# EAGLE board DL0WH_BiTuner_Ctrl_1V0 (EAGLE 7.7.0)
DL0WH Antenna BiTuner
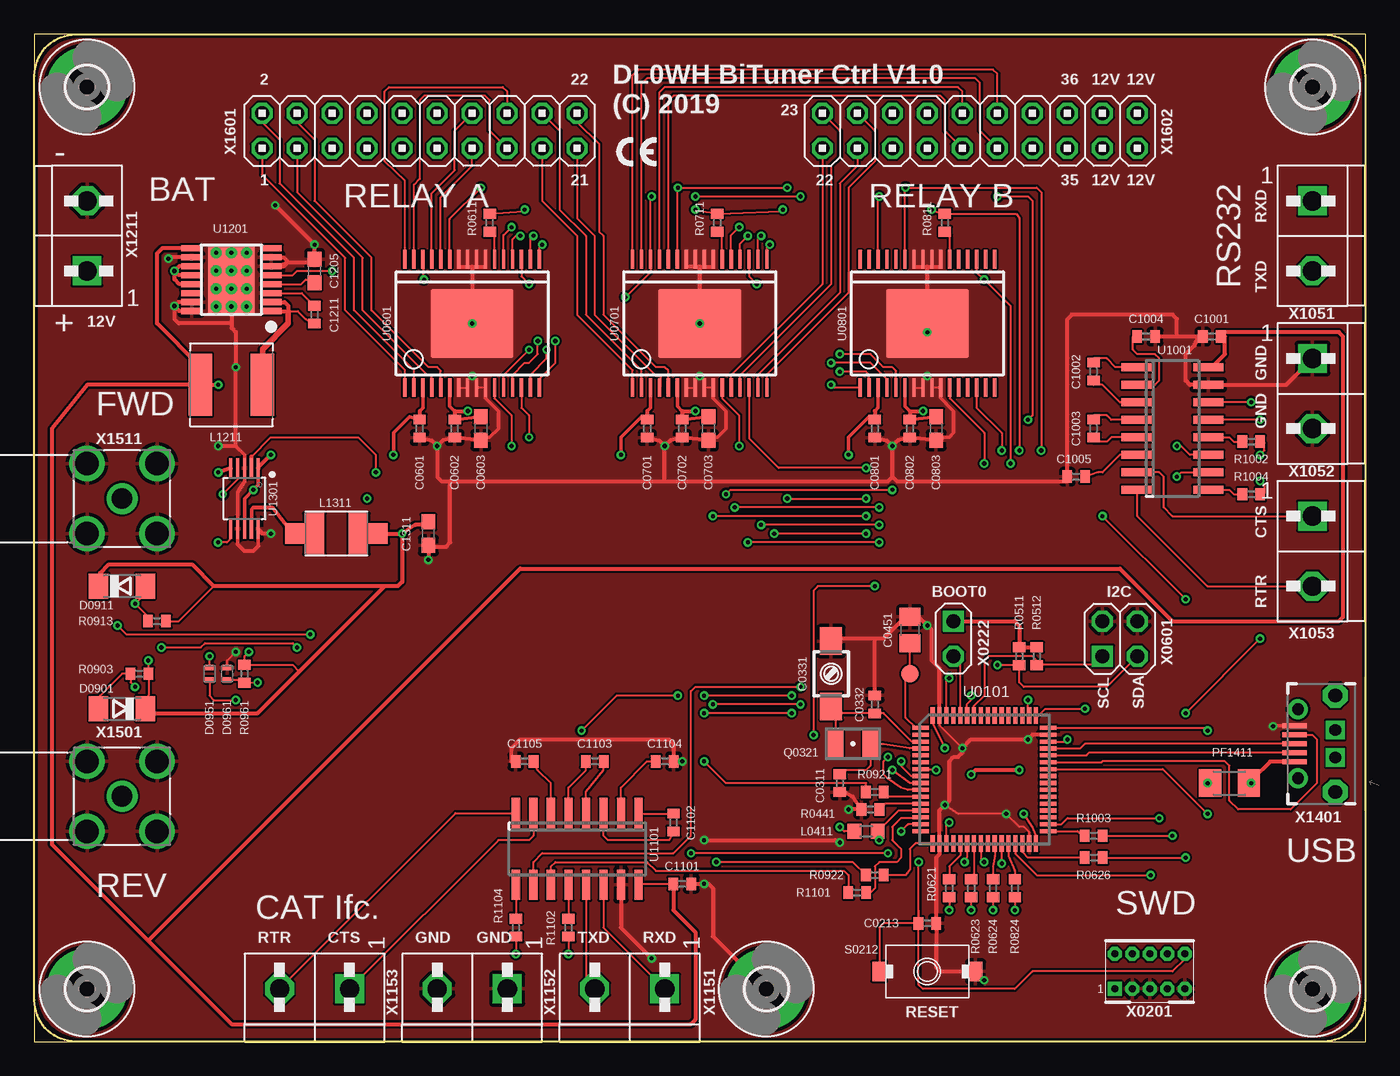
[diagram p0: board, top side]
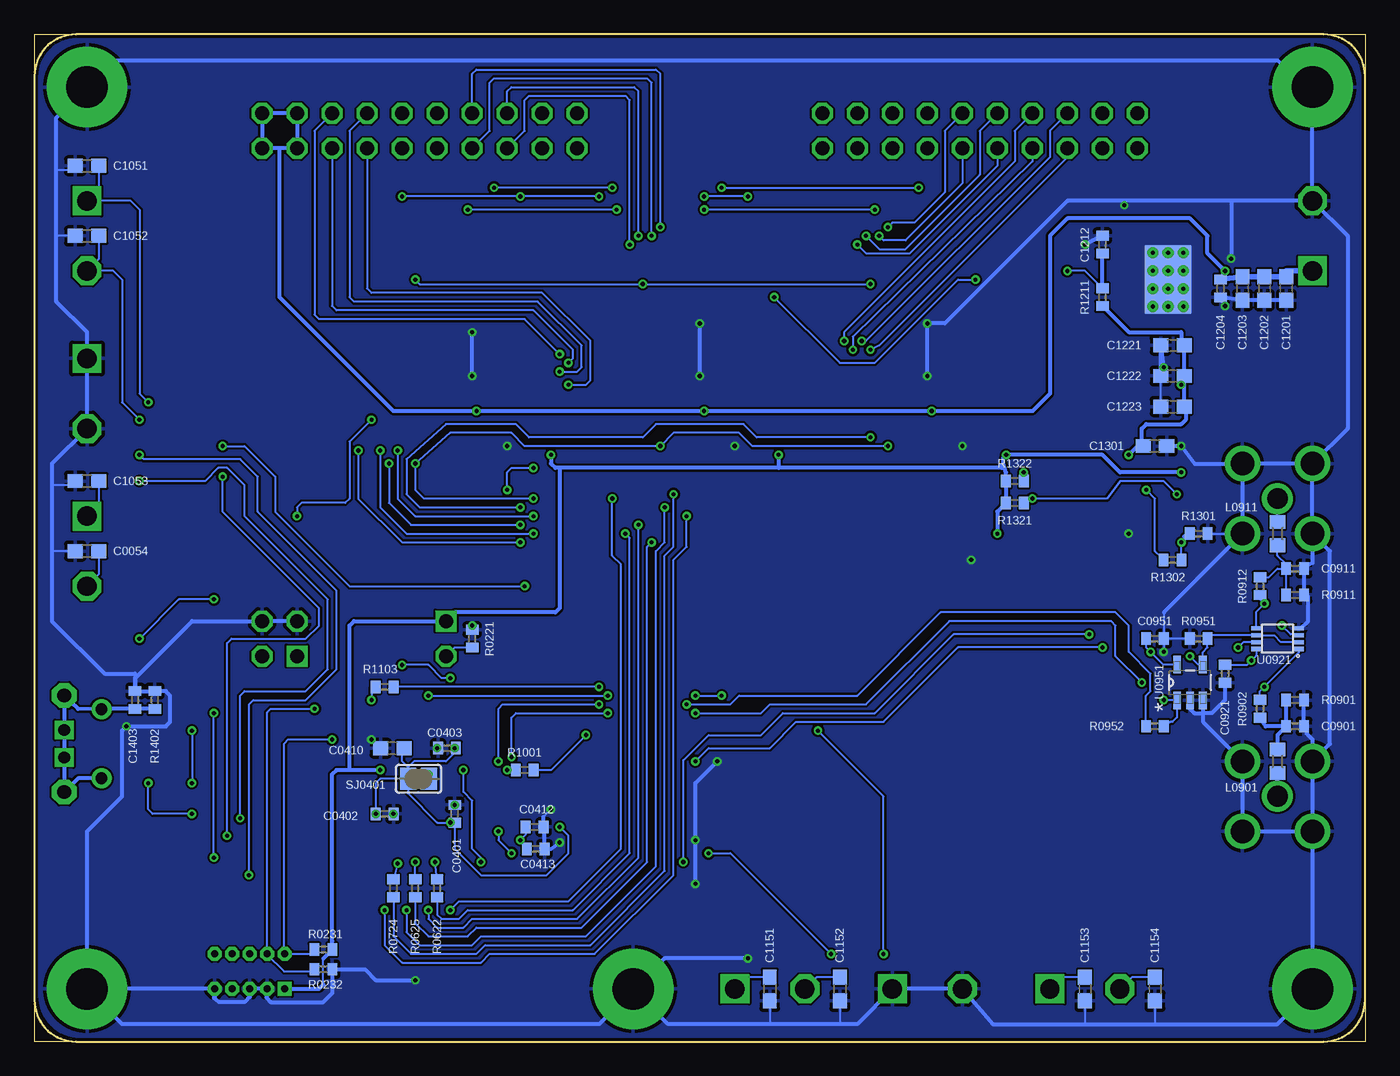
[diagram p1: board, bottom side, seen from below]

Size 96.52 x 73.03 mm. Coordinates in mm from the lower left corner, seen from the top.
Outline: 0,0 96.52,0 96.52,73.03 0,73.03 0,0
Copper layers (1*16): Top 0.035mm / dielectric 1.5mm / Bottom 0.035mm
Design rules "DL0WH_BiTuner_MCU_1V0": minimum track width 6mil, minimum drill 0.3mm, track to track 6mil, track to pad 6mil, pad to pad 6mil, via to via 6mil, smd to smd 0mil, copper to edge 10mil, drill to drill 10mil, minimum pad ring 10mil, minimum via ring 6mil, stop-mask expansion 2mil, vias tented up to drill 25mil, thermal gap 10mil
Net classes: 1 pwr_relay: width 1.5 mm, clearance 0.5 mm; 2 pwr_ttl: width 0.75 mm, clearance 0.5 mm; 3 usb_pair: width 0.254 mm, clearance 0.152 mm; 4 pwrA5: width 0.4 mm; 5 single50R: width 0.838 mm, clearance 0.152 mm
Milling: 8 lines

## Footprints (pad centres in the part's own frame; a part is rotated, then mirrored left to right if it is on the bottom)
C0603 = smd 1.1 x 1: 1 -0.85,0; 2 0.85,0
C0402 = smd 0.7 x 0.9: 1 -0.65,0; 2 0.65,0
3MM2_X_2MM5 = smd 2 x 1.6: + -2.365,0; - 2.365,0
C0805 = smd 1.3 x 1.5: 1 -0.95,0; 2 0.95,0
SOD80C = smd 1.4 x 1.8: A 1.7,0; C -1.7,0
SOD923 = smd 0.4 x 0.6: A 0.45,0; C -0.45,0
3,0-PAD = drill 3 pad 5.842: B3,0 0,0
L0603 = smd 1 x 1.1: 1 -0.85,0; 2 0.85,0
L_6.00MM_X_6.00MM = smd 1.7 x 4.5: 1 -2.25,0; 2 2.25,0
L_4.50MM_X_3.20MM = smd 1.5 x 3: 1 -1.6,0; 2 1.6,0 | smd 2 x 1.5: 3 -2.75,0; 4 2.75,0
M1206 = smd 1.6 x 2: 1 -1.4,0; 2 1.4,0
ABS07 = smd 1.1 x 1.9: 1 -1.25,0; 2 1.25,0
R0402 = smd 0.7 x 0.9: 1 -0.65,0; 2 0.65,0
KSR223G_SMD_1POL = smd 1 x 1.4: 1 -3.5,0; 2 3.5,0
SJ = smd 1.168 x 1.6: 1 -0.762,0; 2 0.762,0
B1,27 = smd 1.27 x 1.27: TP 0,0
LQFP64 = smd 0.3 x 1.2: 1 -3.7,-4.3; 2 -3.2,-4.3; 3 -2.7,-4.3; 4 -2.2,-4.3; 5 -1.7,-4.3; 6 -1.2,-4.3; 7 -0.7,-4.3; 8 -0.2,-4.3; 9 0.3,-4.3; 10 0.8,-4.3; 11 1.3,-4.3; 12 1.8,-4.3; 13 2.3,-4.3; 14 2.8,-4.3; 15 3.3,-4.3; 16 3.8,-4.3; 33 3.8,4.95; 34 3.3,4.95; 35 2.8,4.95; 36 2.3,4.95; 37 1.8,4.95; 38 1.3,4.95; 39 0.8,4.95; 40 0.3,4.95; 41 -0.2,4.95; 42 -0.7,4.95; 43 -1.2,4.95; 44 -1.7,4.95; 45 -2.2,4.95; 46 -2.7,4.95; 47 -3.2,4.95; 48 -3.7,4.95 | smd 1.2 x 0.3: 17 4.675,-3.425; 18 4.675,-2.925; 19 4.675,-2.425; 20 4.675,-1.925; 21 4.675,-1.425; 22 4.675,-0.925; 23 4.675,-0.425; 24 4.675,0.075; 25 4.675,0.575; 26 4.675,1.075; 27 4.675,1.575; 28 4.675,2.075; 29 4.675,2.575; 30 4.675,3.075; 31 4.675,3.575; 32 4.675,4.075; 49 -4.575,4.075; 50 -4.575,3.575; 51 -4.575,3.075; 52 -4.575,2.575; 53 -4.575,2.075; 54 -4.575,1.575; 55 -4.575,1.075; 56 -4.575,0.575; 57 -4.575,0.075; 58 -4.575,-0.425; 59 -4.575,-0.925; 60 -4.575,-1.425; 61 -4.575,-1.925; 62 -4.575,-2.425; 63 -4.575,-2.925; 64 -4.575,-3.425
SOICW32 = smd 0.25 x 1.3: 1 -4.875,-4.65; 2 -4.225,-4.65; 3 -3.575,-4.65; 4 -2.925,-4.65; 5 -2.275,-4.65; 6 -1.625,-4.65; 7 -0.975,-4.65; 8 -0.325,-4.65; 9 0.325,-4.65; 10 0.975,-4.65; 11 1.625,-4.65; 12 2.275,-4.65; 13 2.925,-4.65; 14 3.575,-4.65; 15 4.225,-4.65; 16 4.875,-4.65; 17 4.875,4.65; 18 4.225,4.65; 19 3.575,4.65; 20 2.925,4.65; 21 2.275,4.65; 22 1.625,4.65; 23 0.975,4.65; 24 0.325,4.65; 25 -0.325,4.65; 26 -0.975,4.65; 27 -1.625,4.65; 28 -2.275,4.65; 29 -2.925,4.65; 30 -3.575,4.65; 31 -4.225,4.65; 32 -4.875,4.65 | smd 6 x 5: 33 0,0
R-PDSO-G8 = smd 0.25 x 0.75: 1 -0.75,-1.55; 2 -0.25,-1.55; 3 0.25,-1.55; 4 0.75,-1.55; 5 0.75,1.55; 6 0.25,1.55; 7 -0.25,1.55; 8 -0.75,1.55
SOT-23-5 = smd 1.27 x 0.559: 1 -1.295,0.94; 2 -1.295,0; 3 -1.295,-0.94; 4 1.295,-0.94; 5 1.295,0.94
SOIC16N = smd 0.6 x 2.2: 1 -4.445,-2.6; 2 -3.175,-2.6; 3 -1.905,-2.6; 4 -0.635,-2.6; 5 0.635,-2.6; 6 1.905,-2.6; 7 3.175,-2.6; 8 4.445,-2.6; 9 4.445,2.6; 10 3.175,2.6; 11 1.905,2.6; 12 0.635,2.6; 13 -0.635,2.6; 14 -1.905,2.6; 15 -3.175,2.6; 16 -4.445,2.6
HTSSOP16 = smd 0.45 x 1.5: 1 -2.275,-2.9; 2 -1.625,-2.9; 3 -0.975,-2.9; 4 -0.325,-2.9; 5 0.325,-2.9; 6 0.975,-2.9; 7 1.625,-2.9; 8 2.275,-2.9; 9 2.275,2.9; 10 1.625,2.9; 11 0.975,2.9; 12 0.325,2.9; 13 -0.325,2.9; 14 -0.975,2.9; 15 -1.625,2.9; 16 -2.275,2.9 | drill 0.305 pad 0.61: PAD 0.65,0; PAD3 -0.65,0; PAD4 -1.95,0; PAD5 1.95,0; PAD6 1.95,1.1; PAD7 1.95,-1.1; PAD8 0.65,1.1; PAD9 0.65,-1.1; PAD10 -0.65,1.1; PAD11 -0.65,-1.1; PAD12 -1.95,1.1; PAD13 -1.95,-1.1 | smd 5 x 3.4: PAD1 0,0 | smd 5 x 3.4 bottom: PAD2 0,0
S-PDSO-G10 = smd 0.3 x 1.45: 1 -1,-2.2; 2 -0.5,-2.2; 3 0,-2.2; 4 0.5,-2.2; 5 1,-2.2; 6 1,2.2; 7 0.5,2.2; 8 0,2.2; 9 -0.5,2.2; 10 -1,2.2
2X05_SHROUDED_1MM27 = drill 0.508 pad 0.813 square: 1 -2.54,-1.27 | drill 0.508 pad 0.813 octagon: 2 -2.54,1.27; 3 -1.27,-1.27; 4 -1.27,1.27; 5 0,-1.27; 6 0,1.27; 7 1.27,-1.27; 8 1.27,1.27; 9 2.54,-1.27; 10 2.54,1.27
1X02 = drill 1.016 square: 1 0,0 | drill 1.016 octagon: 2 0,2.54
2X02 = drill 1.016 square: 1 -1.27,-1.27 | drill 1.016 octagon: 2 -1.27,1.27; 3 1.27,-1.27; 4 1.27,1.27
WIRE-TO-BOARD_5MM08_1X02 = drill 1.4 square: 1 0,2.54 | drill 1.4 octagon: 2 0,-2.54
USB-B-MICRO-SMD_MOLEX-105017-0001 = smd 0.35 x 1.8: D+ 0,4.4; D- -0.65,4.4; GND 1.3,4.4; ID 0.65,4.4; VBUS -1.3,4.4 | drill 0.85 pad 1.45: JSHIELD -2.5,4.15; JSHIELD@2 2.5,4.15 | drill 1 pad 1.8 octagon: JSHIELD@3 -3.5,1.45; JSHIELD@6 3.5,1.45 | drill 0.85 square: JSHIELD@4 -1,1.45; JSHIELD@5 1,1.45
SMA_SMT_AMPHENOL_901-143 = drill 1.499: 1 0,0 | drill 1.702: 2 -2.54,2.54; 3 -2.54,-2.54; 4 2.54,-2.54; 5 2.54,2.54
2X10 = drill 1.016 octagon: 1 -11.43,-1.27; 2 -11.43,1.27; 3 -8.89,-1.27; 4 -8.89,1.27; 5 -6.35,-1.27; 6 -6.35,1.27; 7 -3.81,-1.27; 8 -3.81,1.27; 9 -1.27,-1.27; 10 -1.27,1.27; 11 1.27,-1.27; 12 1.27,1.27; 13 3.81,-1.27; 14 3.81,1.27; 15 6.35,-1.27; 16 6.35,1.27; 17 8.89,-1.27; 18 8.89,1.27; 19 11.43,-1.27; 20 11.43,1.27

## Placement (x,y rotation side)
C0054  10nF  [C0603]  92.71,35.56 180 bottom
C0213  100nF  [C0402]  64.77,8.57 0 top
C0311  18pF  [C0402]  58.42,18.73 270 top
C0331  JR200  [3MM2_X_2MM5]  57.78,26.67 270 top
C0332  8.2pF  [C0402]  60.96,24.45 90 top
C0401  100nF  [C0402]  66.04,16.51 90 bottom
C0402  100nF  [C0402]  71.12,16.51 0 bottom
C0403  100nF  [C0402]  66.6,21.27 180 bottom
C0410  4.7uF  [C0603]  70.56,21.27 180 bottom
C0412  10nF  [C0402]  60.25,15.56 0 bottom
C0413  1uF  [C0402]  60.17,13.97 0 bottom
C0451  47uF  [C0805]  63.5,29.84 90 top
C0601  100nF  [C0402]  27.94,44.45 90 top
C0602  100nF  [C0402]  30.48,44.45 270 top
C0603  22uF  [C0603]  32.38,44.45 270 top
C0701  100nF  [C0402]  44.45,44.45 90 top
C0702  100nF  [C0402]  46.99,44.45 270 top
C0703  22uF  [C0603]  48.9,44.45 270 top
C0801  100nF  [C0402]  60.96,44.45 90 top
C0802  100nF  [C0402]  63.5,44.45 270 top
C0803  22uF  [C0603]  65.41,44.45 270 top
C0901  10nF  [C0402]  5.08,22.86 0 bottom
C0911  10nF  [C0402]  5.08,34.29 0 bottom
C0921  100nF  [C0402]  10.16,26.67 270 bottom
C0951  100nF  [C0402]  15.24,29.21 0 bottom
C1001  1uF  [C0402]  85.41,51.12 180 top
C1002  1uF  [C0402]  76.83,48.58 270 top
C1003  1uF  [C0402]  76.83,44.45 270 top
C1004  1uF  [C0402]  80.64,51.12 0 top
C1005  1uF  [C0402]  75.56,40.96 180 top
C1051  10nF  [C0603]  92.71,63.5 180 bottom
C1052  10nF  [C0603]  92.71,58.42 180 bottom
C1053  10nF  [C0603]  92.71,40.64 180 bottom
C1101  1uF  [C0402]  46.99,11.43 0 top
C1102  1uF  [C0402]  46.35,15.88 270 top
C1103  1uF  [C0402]  40.64,20.32 180 top
C1104  1uF  [C0402]  45.72,20.32 0 top
C1105  1uF  [C0402]  35.56,20.32 180 top
C1151  10nF  [C0603]  43.18,3.81 270 bottom
C1152  10nF  [C0603]  38.1,3.81 270 bottom
C1153  10nF  [C0603]  20.32,3.81 270 bottom
C1154  10nF  [C0603]  15.24,3.81 270 bottom
C1201  10uF  [C0603]  5.71,54.61 270 bottom
C1202  10uF  [C0603]  7.3,54.61 270 bottom
C1203  10uF  [C0603]  8.89,54.61 270 bottom
C1204  10nF  [C0402]  10.48,54.61 270 bottom
C1205  3.3uF  [C0603]  20.32,55.88 270 top
C1211  0.47uF  [C0402]  20.32,52.7 90 top
C1212  100nF  [C0402]  19.05,57.78 90 bottom
C1221  22uF  [C0603]  13.97,50.48 180 bottom
C1222  22uF  [C0603]  13.97,48.26 180 bottom
C1223  22uF  [C0603]  13.97,46.04 180 bottom
C1301  22uF  [C0603]  15.24,43.18 0 bottom
C1311  22uF  [C0603]  28.57,36.83 270 top
C1403  1nF  [C0402]  89.22,24.77 270 bottom
D0901  CRS08  [SOD80C]  6.35,24.13 180 top
D0911  CRS08  [SOD80C]  6.35,33.02 0 top
D0951  CMAD6001  [SOD923]  12.7,26.67 90 top
D0961  CMAD6001  [SOD923]  13.97,26.67 270 top
H1711  MOUNT-PAD-ROUND3.0  [3,0-PAD]  3.81,3.81 0 top
H1721  MOUNT-PAD-ROUND3.0  [3,0-PAD]  53.09,3.81 0 top
H1731  MOUNT-PAD-ROUND3.0  [3,0-PAD]  92.71,3.81 0 top
H1751  MOUNT-PAD-ROUND3.0  [3,0-PAD]  3.81,69.22 0 top
H1761  MOUNT-PAD-ROUND3.0  [3,0-PAD]  92.71,69.22 0 top
L0411  10uH  [L0603]  60.33,15.24 0 top
L0901  10uH  [L0603]  6.35,20.32 270 bottom
L0911  10uH  [L0603]  6.35,36.83 90 bottom
L1211  2.2uH  [L_6.00MM_X_6.00MM]  14.29,47.62 0 top
L1311  10uH  [L_4.50MM_X_3.20MM]  21.91,36.83 180 top
PF1411  1.1A/2.2A  [M1206]  86.68,18.73 180 top
Q0321  ABS07-32.768KHZ  [ABS07]  59.37,21.59 180 top
R0221  33kR  [R0402]  64.77,29.21 270 bottom
R0231  220kR  [R0402]  75.56,6.67 0 bottom
R0232  220kR  [R0402]  75.56,5.24 180 bottom
R0441  0R  [R0402]  60.64,16.83 0 top
R0511  1kR  [R0402]  71.44,27.94 90 top
R0512  1kR  [R0402]  72.71,27.94 90 top
R0611  47R  [R0402]  33.02,59.37 270 top
R0621  47R  [R0402]  66.36,11.11 270 top
R0622  0R  [R0402]  67.31,11.11 270 bottom
R0623  47R  [R0402]  67.94,11.11 270 top
R0624  47R  [R0402]  69.53,11.11 270 top
R0625  47R  [R0402]  68.9,11.11 270 bottom
R0626  47R  [R0402]  76.83,13.34 0 top
R0711  47R  [R0402]  49.53,59.37 270 top
R0724  47R  [R0402]  70.48,11.11 270 bottom
R0811  47R  [R0402]  66.04,59.37 270 top
R0824  47R  [R0402]  71.12,11.11 270 top
R0901  1kR  [R0402]  5.08,24.77 180 bottom
R0902  15kR  [R0402]  7.62,24.13 90 bottom
R0903  100kR  [R0402]  7.62,26.67 0 top
R0911  1kR  [R0402]  5.08,32.38 180 bottom
R0912  15kR  [R0402]  7.62,33.02 270 bottom
R0913  100kR  [R0402]  8.89,30.48 0 top
R0921  47R  [R0402]  60.96,18.1 180 top
R0922  47R  [R0402]  60.96,12.06 180 top
R0951  1MR  [R0402]  12.06,29.21 0 bottom
R0952  47R  [R0402]  15.24,22.86 180 bottom
R0961  10kR  [R0402]  15.24,26.67 270 top
R1001  47R  [R0402]  60.96,19.68 0 bottom
R1002  47R  [R0402]  88.27,43.5 180 top
R1003  47R  [R0402]  76.83,14.92 0 top
R1004  47R  [R0402]  88.27,39.69 180 top
R1101  47R  [R0402]  59.69,10.79 180 top
R1102  47R  [R0402]  38.73,8.26 90 top
R1103  47R  [R0402]  71.12,25.72 0 bottom
R1104  47R  [R0402]  34.92,8.26 90 top
R1211  3R  [R0402]  19.05,53.98 270 bottom
R1301  100kR  [R0402]  12.06,36.83 180 bottom
R1302  220kR  [R0402]  13.97,34.92 180 bottom
R1321  1MR  [R0402]  25.4,39.05 180 bottom
R1322  1MR  [R0402]  25.4,40.64 180 bottom
R1402  330kR  [R0402]  87.79,24.77 270 bottom
S0212  KSR223GLFG  [KSR223G_SMD_1POL]  64.77,5.08 180 top
SJ0401  [SJ]  68.66,19.05 180 bottom
TP_VBAT  PTR1B1,27  [B1,27]  63.5,26.67 0 top
U0101  STM32L476RXT_64PIN_LDO  [LQFP64]  68.58,19.05 270 top
U0601  MC33996  [SOICW32]  31.75,52.07 0 top
U0701  MC33996  [SOICW32]  48.26,52.07 0 top
U0801  MC33996  [SOICW32]  64.77,52.07 0 top
U0921  TS5A23166  [R-PDSO-G8]  6.35,29.21 90 bottom
U0951  OPA354  [SOT-23-5]  12.7,26.04 90 bottom
U1001  MAX232_SOIC16  [SOIC16N]  82.55,44.45 270 top
U1101  MAX232_SOIC16  [SOIC16N]  39.37,13.97 180 top
U1201  LM53603-Q1  [HTSSOP16]  14.29,55.24 90 top
U1301  TPS62051  [S-PDSO-G10]  15.24,39.37 180 top
X0201  [2X05_SHROUDED_1MM27]  80.9,5.08 0 top
X0222  [1X02]  66.67,30.48 180 top
X0601  [2X02]  78.74,29.21 0 top
X1051  WIRE-TO-BOARD_5MM08_1X02  [WIRE-TO-BOARD_5MM08_1X02]  92.71,58.42 0 top
X1052  WIRE-TO-BOARD_5MM08_1X02  [WIRE-TO-BOARD_5MM08_1X02]  92.71,46.99 0 top
X1053  WIRE-TO-BOARD_5MM08_1X02  [WIRE-TO-BOARD_5MM08_1X02]  92.71,35.56 0 top
X1151  WIRE-TO-BOARD_5MM08_1X02  [WIRE-TO-BOARD_5MM08_1X02]  43.18,3.81 270 top
X1152  WIRE-TO-BOARD_5MM08_1X02  [WIRE-TO-BOARD_5MM08_1X02]  31.75,3.81 270 top
X1153  WIRE-TO-BOARD_5MM08_1X02  [WIRE-TO-BOARD_5MM08_1X02]  20.32,3.81 270 top
X1211  WIRE-TO-BOARD_5MM08_1X02  [WIRE-TO-BOARD_5MM08_1X02]  3.81,58.42 180 top
X1401  MOLEX 105017-0001  [USB-B-MICRO-SMD_MOLEX-105017-0001]  95.81,21.59 90 top
X1501  SMA_SMT_AMPHENOL-901-143  [SMA_SMT_AMPHENOL_901-143]  6.35,17.78 90 top
X1511  SAMTEC SMA-J-P-H-RA-TH1  [SMA_SMT_AMPHENOL_901-143]  6.35,39.37 90 top
X1601  [2X10]  27.94,66.04 0 top
X1602  [2X10]  68.58,66.04 0 top

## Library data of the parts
C0054 C0213 C0311 C0332 C0401-C0403 C0410 C0412 C0413 C0451 C0601-C0603 C0701-C0703 C0801-C0803 C0901 C0911 C0921 C0951 C1001-C1005 C1051-C1053 C1101-C1105 C1151-C1154 C1201-C1205 C1211 C1212 C1221-C1223 C1301 C1311 C1403 L0411 L0901 L0911 L1211 L1311 R0221 R0231 R0232 R0441 R0511 R0512 R0611 R0621-R0626 R0711 R0724 R0811 R0824 R0901-R0903 R0911-R0913 R0921 R0922 R0951 R0952 R0961 R1001-R1004 R1101-R1104 R1211 R1301 R1302 R1321 R1322 R1402 = df4iah_rcl
C0331 = df4iah_c-trimm
D0901 D0911 D0951 D0961 = df4iah_diode
H1711 H1721 H1731 H1751 H1761 = df4iah_holes
PF1411 = rcl
Q0321 = df4iah_crystal; FARNELL: 2467865; MANUFACTURER: ABS07-32.768KHZ-1-T
S0212 = df4iah_switch
SJ0401 = df4iah_jumper
TP_VBAT = testpad
U0101 = df4iah_stm32l4
U0601 U0701 U0801 = df4iah_dataconvertion
U0921 = df4iah_sc-switches
U0951 = df4iah_opamp; MPN: OPA354AIDBVT; OC_FARNELL: 1207050; OC_NEWARK: -; PACKAGE: SOT-23-5; SUPPLIER: Texas Instruments
U1001 U1101 = df4iah_dataconvertion; MF: MAXIM; MPN: MAX232ECDR; OC_FARNELL: 2463694; OC_NEWARK: unknown
U1201 U1301 = df4iah_powersupply
X0201 X0222 X0601 X1051-X1053 X1151-X1153 X1211 X1401 X1601 X1602 = df4iah_connector
X1501 X1511 = df4iah_connector; MPN: 901-143; OC_FARNELL: 1461631; OC_NEWARK: 51F3841; PACKAGE: RF/COAXIAL, SMA JACK, R/A, 50OHM, THD; SUPPLIER: Amphenol

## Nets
+3V3: C0601.2 C0701.2 C0801.2 C0921.1 C0951.1 C1311.1 D0901.C D0911.C L1311.1 L1311.3 R0231.2 R0511.2 R0512.2 R0903.2 R0913.2 R0961.1 R1321.2 R1322.2 SJ0401.1 U0601.3 U0701.3 U0801.3 U0921.8 U0951.5 U1301.5 X0201.1 X0222.1
+5V: C1001.1 C1101.1 C1221.1 C1222.1 C1223.1 C1301.1 L1211.1 R1211.2 R1302.2 U1001.16 U1101.16 U1201.9 U1301.1 U1301.8
+12V: C0602.1 C0603.1 C0702.1 C0703.1 C0802.1 C0803.1 C1201.1 C1202.1 C1203.1 C1204.1 U0601.6 U0701.6 U0801.6 U1201.11 U1201.12 U1201.13 X1211.1 X1602.17 X1602.18 X1602.19 X1602.20
CAT_DTE_CTS: C1153.1 U1101.7 X1153.1
CAT_DTE_RTR: C1154.1 U1101.8 X1153.2
CAT_DTE_RXD: C1151.1 U1101.14 X1151.1
CAT_DTE_TXD: C1152.1 U1101.13 X1151.2
CAT_MX_C1N: C1102.2 U1101.3
CAT_MX_C1P: C1102.1 U1101.1
CAT_MX_C2M: C1103.2 U1101.5
CAT_MX_C2P: C1103.1 U1101.4
CAT_MX_VM: C1105.1 U1101.6
CAT_MX_VP: C1104.1 U1101.2
DRV_OUT_3_4: U0801.12
DRV_OUT_3_5: U0801.13
DRV_OUT_3_6: U0801.15
DRV_OUT_3_7: U0801.16
DRV_OUT_3_8: U0801.17
DRV_OUT_3_9: U0801.18
DRV_OUT_3_10: U0801.20
DRV_OUT_3_11: U0801.21
DRV_OUT_3_12: U0801.28
DRV_OUT_3_13: U0801.29
DRV_OUT_3_14: U0801.31
DRV_OUT_3_15: U0801.32
GND: C0054.2 C0213.2 C0311.2 C0331.+ C0332.2 C0401.2 C0402.2 C0403.2 C0410.2 C0412.2 C0413.2 C0451.2 C0601.1 C0602.2 C0603.2 C0701.1 C0702.2 C0703.2 C0801.1 C0802.2 C0803.2 C0901.2 C0911.2 C0921.2 C0951.2 C1001.2 C1004.2 C1005.2 C1051.2 C1052.2 C1053.2 C1101.2 C1104.2 C1105.2 C1151.2 C1152.2 C1153.2 C1154.2 C1201.2 C1202.2 C1203.2 C1204.2 C1205.1 C1212.2 C1221.2 C1222.2 C1223.2 C1301.2 C1311.2 C1403.1 D0961.C H1711.B3,0 H1721.B3,0 H1731.B3,0 H1751.B3,0 H1761.B3,0 R0221.1 R0232.1 R0441.1 R0901.1 R0911.1 R0951.1 R1301.1 R1402.1 S0212.1 U0101.18 U0101.31 U0101.47 U0101.63 U0601.7 U0601.8 U0601.9 U0601.10 U0601.23 U0601.24 U0601.25 U0601.26 U0601.33 U0701.7 U0701.8 U0701.9 U0701.10 U0701.23 U0701.24 U0701.25 U0701.26 U0701.33 U0801.7 U0801.8 U0801.9 U0801.10 U0801.23 U0801.24 U0801.25 U0801.26 U0801.33 U0921.4 U0951.2 U0951.3 U1001.15 U1101.15 U1201.6 U1201.7 U1201.10 U1201.15 U1201.16 U1201.PAD U1201.PAD1 U1201.PAD2 U1201.PAD3 U1201.PAD4 U1201.PAD5 U1201.PAD6 U1201.PAD7 U1201.PAD8 U1201.PAD9 U1201.PAD10 U1201.PAD11 U1201.PAD12 U1201.PAD13 U1301.3 U1301.7 U1301.10 X0201.3 X0201.5 X0201.9 X0601.2 X0601.4 X1052.1 X1052.2 X1152.1 X1152.2 X1211.2 X1401.GND X1501.2 X1501.3 X1501.4 X1501.5 X1511.2 X1511.3 X1511.4 X1511.5
LM53603_!RESET: U1201.8
LM53603_BIAS: C1212.1 R1211.1 U1201.5
LM53603_CBOOT: C1211.2 U1201.3
LM53603_SW: C1211.1 L1211.2 U1201.1 U1201.2
LM53603_VCC: C1205.2 U1201.4
MCU_NRST: C0213.1 S0212.2 U0101.7 X0201.10
MCU_VBAT: C0451.1 TP_VBAT.TP U0101.1
MCU_VDD: C0401.1 C0402.1 C0403.1 C0410.1 L0411.1 SJ0401.2 U0101.19 U0101.32 U0101.64
MCU_VDDA: C0412.1 C0413.1 L0411.2 U0101.13
MCU_VREF_M: R0441.2 U0101.12
MP_CAT_CTS_R: R1103.2 U1101.10
MP_CAT_RTR_R: R1104.2 U1101.9
MP_CAT_RXD_R: R1101.2 U1101.11
MP_CAT_TXD_R: R1102.2 U1101.12
MP_RS_CTS_R: R1003.2 U1001.10
MP_RS_RTR_R: R1004.2 U1001.9
MP_RS_RXD_R: R1001.2 U1001.11
MP_RS_TXD_R: R1002.2 U1001.12
N$12: R0611.2 U0601.22
N$13: R0711.2 U0701.22
N$15: R0811.2 U0801.22
PA0: R1101.1 U0101.14
PA1: R1102.1 U0101.15
PA2: U0101.16
PA3: R0922.1 U0101.17
PA4: U0101.20
PA5: R0621.1 U0101.21
PA6: R0622.1 U0101.22
PA7: R0623.1 U0101.23
PA8: U0101.41
PA9: PF1411.1 U0101.42 X1401.VBUS
PA10: U0101.43 X1401.ID
PA11: U0101.44 X1401.D-
PA12: U0101.45 X1401.D+
PA13: R0231.1 U0101.46 X0201.2
PA14: R0232.2 U0101.49 X0201.4
PA15: R1103.1 U0101.50
PB0: R0624.1 U0101.26
PB1: R0724.1 U0101.27
PB2: R0824.1 U0101.28
PB3: U0101.55
PB4: U0101.56
PB5: U0101.57
PB6: R0512.1 U0101.58 X0601.1
PB7: R1104.1 U0101.59
PB8: U0101.61
PB9: R0511.1 U0101.62 X0601.3
PB10: R1002.1 U0101.29
PB11: R0626.1 U0101.30
PB12: R1003.1 U0101.33
PB13: R1004.1 U0101.34
PB14: U0101.35
PB15: U0101.36
PC0: R0952.2 U0101.8
PC1: R1001.1 U0101.9
PC2: D0961.A R0961.2 U0101.10
PC3: R0921.1 U0101.11
PC4: R0625.1 U0101.24
PC5: U0101.25
PC6: U0101.37
PC7: U0101.38
PC8: U0101.39
PC9: U0101.40
PC10: U0101.51
PC11: U0101.52
PC12: U0101.53
PC13: U0101.2
PC14_OSC32_IN: C0331.- C0332.1 Q0321.2 U0101.3
PC15_OSC32_OUT: C0311.1 Q0321.1 U0101.4
PD2: U0101.54
PH0: U0101.5
PH1: U0101.6
PH3_BOOT0: R0221.2 U0101.60 X0222.2
RELAY1: U0601.1 X1601.1
RELAY2: U0601.2 X1601.2
RELAY3: U0601.4 X1601.3
RELAY4: U0601.5 X1601.4
RELAY5: U0601.12 X1601.5
RELAY6: U0601.13 X1601.6
RELAY7: U0601.15 X1601.7
RELAY8: U0601.16 X1601.8
RELAY9: U0601.17 X1601.9
RELAY10: U0601.18 X1601.10
RELAY11: U0601.20 X1601.11
RELAY12: U0601.21 X1601.12
RELAY13: U0601.28 X1601.13
RELAY14: U0601.29 X1601.14
RELAY15: U0601.31 X1601.15
RELAY16: U0601.32 X1601.16
RELAY17: U0701.1 X1601.17
RELAY18: U0701.2 X1601.18
RELAY19: U0701.4 X1601.19
RELAY20: U0701.5 X1601.20
RELAY21: U0701.12 X1602.1
RELAY22: U0701.13 X1602.2
RELAY23: U0701.15 X1602.3
RELAY24: U0701.16 X1602.4
RELAY25: U0701.17 X1602.5
RELAY26: U0701.18 X1602.6
RELAY27: U0701.20 X1602.7
RELAY28: U0701.21 X1602.8
RELAY29: U0701.28 X1602.9
RELAY30: U0701.29 X1602.10
RELAY31: U0701.31 X1602.11
RELAY32: U0701.32 X1602.12
RELAY33: U0801.1 X1602.13
RELAY34: U0801.2 X1602.14
RELAY35: U0801.4 X1602.15
RELAY36: U0801.5 X1602.16
RM_FWD: L0901.2 X1501.1
RM_REV: L0911.2 X1511.1
RS_DTE_CTS: C1053.1 U1001.7 X1053.1
RS_DTE_RTR: C0054.1 U1001.8 X1053.2
RS_DTE_RXD: C1051.1 U1001.14 X1051.1
RS_DTE_TXD: C1052.1 U1001.13 X1051.2
RS_MX_C1N1: C1002.2 U1001.3
RS_MX_C1P: C1002.1 U1001.1
RS_MX_C2M1: C1003.2 U1001.5
RS_MX_C2P: C1003.1 U1001.4
RS_MX_VM: C1005.1 U1001.6
RS_MX_VP: C1004.1 U1001.2
SPI_DRV_!RST: R0625.2 U0601.27 U0701.27 U0801.27
SPI_DRV_C_!CS: R0724.2 U0701.14
SPI_DRV_EXT_!CS: R0824.2 U0801.14
SPI_DRV_L_!CS: R0624.2 U0601.14
SPI_DRV_PWM: R0626.2 U0601.30 U0701.30 U0801.30
SPI_DRV_SCLK: R0621.2 U0601.11 U0701.11 U0801.11
SPI_DRV_SI: R0623.2 U0601.19 U0701.19 U0801.19
SPI_DRV_SO: R0611.1 R0622.2 R0711.1 R0811.1
SWR_IN_FWD: D0901.A R0902.2 R0903.1 U0921.1
SWR_IN_FWD_HI: C0901.1 L0901.1 R0901.2 R0902.1
SWR_IN_REV: D0911.A R0912.2 R0913.1 U0921.5
SWR_IN_REV_HI: C0911.1 L0911.1 R0911.2 R0912.1
SWR_OP_OUT: D0951.C R0952.1 U0951.1
SWR_SEL_FWD: R0921.2 U0921.7
SWR_SEL_PWR: D0951.A R0951.2 U0921.2 U0921.6 U0951.4
SWR_SEL_REV: R0922.2 U0921.3
TPS_LBI: R1301.2 R1302.1 U1301.6
TPS_LBO: R1322.1 U1301.2
TPS_PG: R1321.1 U1301.4
TPS_SW: L1311.2 L1311.4 U1301.9
USB_SHIELD: C1403.2 R1402.2 X1401.JSHIELD X1401.JSHIELD@2 X1401.JSHIELD@3 X1401.JSHIELD@4 X1401.JSHIELD@5 X1401.JSHIELD@6
VDDUSB: PF1411.2 U0101.48

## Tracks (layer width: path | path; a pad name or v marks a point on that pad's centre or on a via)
+3V3  (via drill 0.3)
  Top 0.152: R0913.2 10.48,30.48 13.02,33.02 | 19.21,26.83 18.72,27.32 R0961.1 15.24,27.94 v15.56,28.26 | D0901.C 8.26,24.34 8.26,25.08 8.27,25.1 R0903.2 8.27,27.61 v8.26,27.62 | D0911.C 4.76,33.02
  Top 0.254: U0601.3 28.18,45.95 27.94,45.72 | U0701.3 44.69,45.95 44.45,45.72 | U0801.3 61.2,45.95 60.96,45.72 | C0601.2 27.2,45.3 26.04,44.13 v26.04,42.55 | C0701.2 44.03,45.3 42.55,43.81 v42.55,42.55 | C0801.2 60.54,45.3 59.05,43.81 v59.05,42.55
  Top 0.305: C1311.1 28.26,37.47 27.62,37.47 v26.67,36.83 | L1311.1 L1311.3 v26.67,36.83 | U1301.5 13.29,41.23 v13.34,41.27 | 27.94,45.72 C0601.2 | 44.45,45.72 C0701.2 | 60.96,45.72 C0801.2 | X0222.1 71.12,30.48 71.44,30.16 R0511.2 R0512.2 | v71.44,19.68 68.26,19.68 v67.94,19.37 | v26.67,36.83 26.67,33.34 26.35,33.02 25.4,33.02 | 25.4,33.02 13.02,33.02 11.43,34.61 5.4,34.61 4.76,33.97 4.76,33.02 | 7.94,24.13 D0901.C 8.57,23.81 16.19,23.81 19.21,26.83 25.4,33.02
  Bottom 0.152: 75.56,4.13 75.56,6.02 | v67.94,19.37 67.94,19.1 SJ0401.1 | C0951.1 15.89,28.59 v15.56,28.26 14.63,27.33 U0951.5 | U0921.8 7.9,27.98 v8.26,27.62 8.56,27.32 C0921.1
  Bottom 0.305: v26.67,36.83 26.67,38.42 R1321.2 R1322.2 26.04,41.27 26.25,41.91 | v13.34,41.27 17.78,41.27 19.05,42.55 v26.04,42.55 26.25,42.33 26.25,41.91 | v59.05,42.55 59.05,41.91 58.74,41.59 58.42,41.59 | 26.25,41.91 26.35,41.81 26.35,41.59 42.55,41.59 | X0201.1 75.88,3.81 75.56,4.13 | 75.56,6.02 R0231.2 74.92,7.29 74.93,9.21 74.93,19.37 74.61,19.68 73.66,19.68 | v71.44,19.68 73.66,19.68 | 73.66,19.68 73.66,30.16 73.34,30.48 X0222.1 66.04,31.11 58.74,31.11 58.42,31.43 58.42,41.27 58.42,41.59 | 42.55,41.59 58.42,41.59 | v42.55,42.55 42.55,41.59
+5V  (via drill 0.3)
  Top 0.152: U1101.16 43.88,11.43 C1101.1 | 11.75,47.62 L1211.1
  Top 0.254: U1301.1 16.24,40.37 v15.88,40.01 15.24,39.37 U1301.8
  Top 0.305: U1201.9 9.26,57.52 8.89,57.15 8.89,52.07 12.04,48.92 L1211.1 v13.34,47.62 | U1301.1 16.24,41.64 v17.14,42.55 | 11.75,47.62 3.81,47.62 1.27,44.45 1.27,14.29 8.26,7.3 | 8.26,7.3 14.29,1.27 47.62,1.27 47.94,1.59 47.94,7.94 46.35,9.53 46.35,11.12 C1101.1 | 8.26,7.3 35.24,34.29 78.74,34.29 82.55,30.48 94.61,30.48 94.93,30.8 94.93,51.12 94.61,51.44 86.38,51.44 C1001.1 86.36,51.12 86.36,49.85 85.41,48.9 U1001.16
  Bottom 0.152: 14.82,35.14 15.24,35.56 15.24,39.37 v15.88,40.01
  Bottom 0.305: C1222.1 C1223.1 13,45.73 13.02,45.09 13.34,44.77 15.88,44.77 16.19,44.45 16.19,43.5 C1301.1 16.51,43.18 v17.14,42.55 | C1222.1 C1221.1 13.34,50.5 13.34,51.44 17.14,51.44 19.04,53.33 R1211.2 | C1222.1 13.32,47.64 v13.34,47.62 | R1302.2 14.82,35.14
+12V  (via drill 0.3)
  Top 0.254: U0601.6 30.12,46.08 30.48,45.72 | C0603.1 C0602.1 | U0701.6 46.63,46.08 46.99,45.72 | C0703.1 C0702.1 | U0801.6 63.15,46.08 63.5,45.72 | C0803.1 C0802.1
  Top 0.305: C0602.1 30.48,45.72 v31.43,45.72 | C0702.1 46.99,45.72 v47.94,45.72 | C0802.1 63.5,45.72 v64.45,45.72 | U1201.11 10.5,56.22 v10.16,55.88 | U1201.12 10.47,55.57 v10.16,55.88 | U1201.13 10.5,54.92 10.16,55.26 v10.16,55.88
  Bottom 0.305: 7.62,55.24 C1202.1 | C1204.1 v10.16,55.88 11.43,57.15 11.43,58.42 12.7,59.69 21.59,59.69 22.86,58.42 22.86,46.99 24.13,45.72 v31.43,45.72 v47.94,45.72 v64.45,45.72 70.48,45.72 78.74,53.98 78.74,64.77 | 78.74,64.77 X1602.17 X1602.18 X1602.20 X1602.19 78.74,64.77
  Bottom 0.406: C1204.1 C1203.1 C1202.1 C1201.1 5.73,55.88 X1211.1
CAT_DTE_CTS
  Top 0.152: X1153.1 33.66,14.61 35.88,14.61 36.2,14.92 U1101.7
  Bottom 0.152: C1153.1 22.01,4.66 X1153.1
CAT_DTE_RTR
  Top 0.152: X1153.2 30.54,16.57 U1101.8
  Bottom 0.152: C1154.1 16.93,4.66 X1153.2
CAT_DTE_RXD
  Top 0.152: U1101.14 41.27,8.26 X1151.1
  Bottom 0.152: C1151.1 44.87,4.66 X1151.1
CAT_DTE_TXD
  Top 0.152: U1101.13 40.01,4.45 X1151.2
  Bottom 0.152: C1152.1 39.79,4.66 X1151.2
CAT_MX_C1N
  Top 0.152: C1102.2 46.04,14.61 41.59,14.61 41.27,14.92 U1101.3
CAT_MX_C1P
  Top 0.152: U1101.1 44.2,16.51 C1102.1
CAT_MX_C2M
  Top 0.152: U1101.5 38.73,18.41 40.01,19.69 C1103.2
CAT_MX_C2P
  Top 0.152: U1101.4 40.01,18.1 41.27,19.68 C1103.1
CAT_MX_VM
  Top 0.152: U1101.6 37.47,18.73 36.51,19.69 C1105.1
CAT_MX_VP
  Top 0.152: U1101.2 42.55,18.41 44.45,20.32 C1104.1
GND  (via drill 0.3)
  Top 0.152: U0601.7 U0601.8 31.43,47.94 v31.75,48.26 32.08,47.94 U0601.9 U0601.10 | U0701.7 U0701.8 47.94,47.94 v48.26,48.26 48.59,47.94 U0701.9 U0701.10 | U0801.7 U0801.8 64.44,47.94 v64.77,48.26 65.09,47.94 U0801.9 U0801.10 65.75,46.7 65.72,46.67 | 32.7,56.2 32.7,56.7 U0601.23 | 30.8,56.2 30.8,56.7 U0601.26 | U0601.25 31.43,56.2 | U0601.24 32.08,56.2 32.07,56.2 | U0801.26 63.8,56.22 63.82,56.2 | U0801.25 64.44,56.2 64.45,56.2 | U0801.24 65.09,56.2 | U0801.23 65.75,56.22 65.72,56.2 | S0212.1 | 58.74,18.1 58.72,18.1 C0311.2 | U0101.31 72.16,15.16 71.75,15.56 71.44,15.56 v70.48,16.51 66.99,16.51 v66.04,17.14 | U0101.63 65.66,22.93 v67.31,21.27 | R0441.1 59.69,16.83 | 53.02,3.87 H1721.B3,0 53.02,3.81 | 84.45,51.12 C1001.2 | 64.14,30.8 C0451.2 63.18,30.8 | 57.96,29.21 C0331.+ | C0803.2 65.83,43.6 66.04,43.81 | D0961.C 13.97,27.62 v14.61,28.26
  Top 0.254: 14.61,43.18 15.24,42.55 U1301.3 15.24,40.64 14.74,39.82 U1301.7 14.74,36.06 | U1301.10 16.24,35.92 | U0701.10 49.23,46.65 50.16,45.72 50.16,44.45 49.53,43.81 49.11,43.81 C0703.2 | 32.49,43.6 C0603.2 32.6,43.81 33.02,43.81 33.66,44.45 33.66,45.72 32.73,46.65 U0601.10 | U0701.26 47.28,56.22 47.31,56.2 | U0701.23 49.23,56.22 49.21,56.2 | U0701.25 47.94,56.2 | U0701.24 48.59,56.2 48.58,56.2 | X1401.GND 89.88,22.89 v89.85,22.86 | 65.72,43.81 66.04,43.81 66.36,43.81 66.67,44.13 66.67,45.72 65.72,46.67
  Top 0.305: U1201.10 9.88,56.87 v9.72,56.77 | U1201.6 17.78,56.22 | 17.78,56.22 18.12,56.22 18.41,56.52 | 18.41,56.52 20.3,56.52 C1205.1 v20.32,57.78 v17.46,60.64 | U1201.7 18.06,56.87 18.41,56.52 | 18.41,56.52 17.78,56.22 | U1201.15 10.44,53.62 v10.16,53.34 | U1201.16 10.53,52.97 v10.16,53.34 | v13.34,43.18 14.61,43.18 v14.61,48.9 14.61,51.44 14.29,51.75 14.29,52.07 | 16.24,35.92 15.88,35.56 15.24,35.56 14.74,36.06 | v17.14,36.83 16.51,36.83 16.51,36.9 U1301.10 | C0601.1 28.79,43.6 v29.21,43.18 | C0603.2 C0602.2 29.63,43.6 v29.21,43.18 | v28.57,34.92 C1311.2 28.89,35.88 29.84,35.88 30.16,36.2 30.16,40.64 | C0701.1 45.3,43.6 v45.72,43.18 | v45.72,43.18 46.14,43.6 C0702.2 C0703.2 | C0803.2 C0802.2 62.65,43.6 v62.23,43.18 | C0801.1 61.81,43.6 v62.23,43.18 | U1201.PAD4 14.29,52.07 | 14.29,52.07 10.48,52.07 10.16,52.39 v10.16,53.34 | v29.21,43.18 29.21,40.96 29.53,40.64 30.16,40.64 | 30.16,40.64 45.72,40.64 | 45.72,40.64 61.91,40.64 62.23,40.96 | 62.23,40.96 v62.23,43.18 | 45.72,40.64 v45.72,43.18 | 30.8,56.2 31.43,56.2 31.75,56.2 | 31.75,56.2 32.07,56.2 32.7,56.2 | 31.75,56.2 U0601.33 | U0701.33 48.26,56.2 | 48.26,56.2 47.94,56.2 47.31,56.2 | 48.26,56.2 48.58,56.2 49.21,56.2 | 63.82,56.2 64.45,56.2 64.77,56.2 | 64.77,56.2 65.09,56.2 65.72,56.2 | v64.77,51.44 U0801.33 64.77,56.2 | S0212.1 65.72,5.08 65.41,5.4 C0213.2 65.41,9.12 65.41,13.34 65.66,13.59 U0101.18 65.66,16.76 v66.04,17.14 66.36,17.46 66.36,20.32 66.67,20.64 66.99,20.64 67.31,20.95 v67.31,21.27 67.94,21.91 v72.07,21.91 72.42,22.25 U0101.47 | S0212.1 v68.9,4.45 | R0441.1 59.36,17.77 58.74,18.1 | 59.69,16.83 v59.05,16.83 | 53.02,3.87 49.21,7.62 49.21,11.11 48.9,11.43 v48.58,11.43 C1101.2
  Top 0.305: U1101.15 42.55,8.26 v44.77,6.03 | C1105.2 34.61,20.32 34.61,21.27 35.24,21.91 46.04,21.91 46.35,21.59 46.35,21.27 C1104.2 v46.99,20.32 | X1052.1 90.81,47.62 U1001.15 83.82,47.62 83.5,47.94 83.5,49.85 84.14,50.48 84.45,51.12 | 62.23,40.96 62.55,40.64 74.93,40.64 74.93,40.95 C1005.2 74.93,52.39 75.25,52.7 82.55,52.7 82.87,52.39 82.87,51.12 | C1001.2 82.87,51.12 | 82.87,51.12 C1004.2 | 64.14,30.8 v64.77,30.16 65.09,29.84 65.09,27.62 65.66,27.05 U0101.63 | 63.18,30.8 61.59,29.21 60.96,29.21 | 60.96,29.21 57.96,29.21 | C0332.2 60.96,29.21 | v48.58,14.61 58.07,14.61 v58.42,14.43
  Bottom 0.152: R1301.1 X1511.3 | C1223.2 C1222.2 | X0201.3 79.69,3.81 | 59.52,15.48 C0412.2 | C0410.2 71.44,21.27 v72.07,21.91 | C0402.2 70.47,16.21 v70.48,16.51 | C0401.2 66.34,17.16 v66.04,17.14 | C0403.2 67.25,21.53 v67.31,21.27 | 59.6,16.29 v59.05,16.83 | R0221.1 v64.77,30.16 | 83.5,3.81 X0201.9 | R0951.1 C0951.2 | 14.59,31.11 C0951.2 | C0951.2 14.59,28.27 v14.61,28.26 | C1152.2 38.1,1.27 | C1151.2 43.18,1.27 | C1154.2 15.24,1.27 | C1153.2 20.32,1.27 | C1051.2 93.88,63.18 94.93,63.18 | C1052.2 94.93,58.42 | C1053.2 93.88,40.32 95.25,40.32 | C0054.2 95.25,35.56
  Bottom 0.305: C1212.2 20.3,57.8 v20.32,57.78 | v10.16,53.34 C1204.2 C1203.2 C1202.2 C1201.2 | C1301.2 v13.34,43.18 12.38,41.91 X1511.4 | X1211.2 9.72,60.96 | 9.72,60.96 v9.72,56.77 | X1211.2 H1751.B3,0 6.35,71.12 90.81,71.12 H1761.B3,0 94.93,66.99 94.93,63.18 94.93,58.42 94.93,53.66 92.71,51.44 X1052.1 X1052.2 95.25,41.91 95.25,40.32 95.25,35.56 95.25,30.48 91.44,26.67 89.22,26.67 C1403.1 89.2,25.4 C1403.1 | X1501.2 H1711.B3,0 6.35,1.27 15.24,1.27 20.32,1.27 26.99,1.27 X1152.2 X1152.1 36.83,1.27 38.1,1.27 43.18,1.27 50.55,1.27 H1721.B3,0 | X1501.2 X1501.3 X1501.4 11.76,23.19 11.76,23.81 | X1501.5 X1501.2 | X1501.5 3.81,21.91 4.23,22.33 C0901.2 R0901.1 | U0951.3 11.76,23.81 | U0951.2 12.7,24.13 12.38,23.81 11.76,23.81 | C0921.2 10.16,24.77 11.11,23.81 11.76,23.81 | X1511.2 3.81,34.71 C0911.2 R0911.1 4.13,32.28 4.13,30.48 4.65,29.96 U0921.4 | X1511.5 X1511.4 | X1511.2 X1511.5 | X1511.4 X1511.3 14.45,31.27 14.59,31.11 | C1222.2 C1221.2 v14.62,48.91 v14.61,48.9 | X1211.2 1.27,58.42 1.27,44.45 X1511.5 | 9.72,60.96 17.46,60.96 | 17.46,60.96 21.59,60.96 30.48,52.07 U0601.33 v31.75,48.26 | v17.46,60.64 17.46,60.96 | v48.26,48.26 U0701.33 | v64.77,48.26 v64.77,51.44 | H1731.B3,0 92.71,15.24 90.17,17.78 90.17,22.54 v89.85,22.86 87,22.86 86.68,23.18 86.68,25.08 87,25.4 87.77,25.4 R1402.1 C1403.1 | 83.5,3.81 H1731.B3,0 | v68.9,4.45 71.75,4.45 72.55,5.24 R0232.1 74.92,3.51 75.56,2.86 79.38,2.86 79.69,3.17 79.69,3.81 X0201.5 80.9,3.24 81.28,2.86 83.12,2.86 83.5,3.17 83.44,3.24 X0201.9 | 59.52,15.48 C0413.2 59.05,13.97 v58.42,14.43 | X0601.2 X0601.4 85.09,30.48 89.22,26.35 C1403.1 | C0412.2 59.6,16.29
  Bottom 0.305: v44.77,6.03 50.8,6.03 55.56,1.27 90.17,1.27 H1731.B3,0 | v48.58,11.43 v48.58,14.61 48.58,18.73 v46.99,20.32 | X1501.5 2.54,21.59 2.54,35.56 X1511.2
  other vias: 31.75,52.07 48.26,52.07
  pour Top: 0.32,3.32 0.32,69.71 arc-88 3,72.71 93.2,72.71 arc-98 96.2,69.71 96.2,3.32 arc-88 93.2,0.32 3,0.32 arc-78
  pour Bottom: 0.32,3.32 0.32,69.71 arc-88 3,72.71 93.2,72.71 arc-98 96.2,69.71 96.2,3.32 arc-88 93.2,0.32 3,0.32 arc-78
LM53603_BIAS  (via drill 0.3)
  Top 0.152: U1201.5 18.74,55.57 19.05,55.88 v21.59,55.88
  Bottom 0.152: R1211.1 19.7,55.26 20.32,55.88 v21.59,55.88
  Bottom 0.305: R1211.1 C1212.1
LM53603_CBOOT
  Top 0.152: U1201.3 19.39,54.27 20,53.66 20.3,53.34
  Top 0.305: 20.3,53.34 C1211.2
LM53603_SW
  Top 0.152: 18.41,52.97 19.1,52.97 19.68,52.39 20.3,52.07
  Top 0.305: U1201.1 18.41,52.97 18.41,53.34 18.14,53.62 U1201.2 | 20.3,52.07 C1211.1
  Top 0.406: L1211.2 16.54,50.19 18.41,52.07 18.41,52.97
LM53603_VCC
  Top 0.152: U1201.4 19.36,54.92 19.68,55.24 20.3,55.24
  Top 0.305: 20.3,55.24 C1205.2
MCU_NRST  (via drill 0.3)
  Top 0.152: C0213.1 61.59,8.57 61.28,8.26 S0212.2 | X0201.10 83.44,5.97 82.55,5.08 72.39,5.08 71.12,3.81 64.45,3.81 64.14,4.13 64.14,9.51 C0213.1 | U0101.7 65.34,19.75 v65.41,19.68 | C0213.1 64.12,10.46 v64.14,13.02
  Bottom 0.152: v64.14,13.02 64.14,13.34 64.77,13.97 64.77,17.46 65.41,18.1 v65.41,19.68
MCU_VBAT
  Top 0.152: U0101.1 63.93,22.75 63.18,23.5 63.18,26.99 TP_VBAT.TP C0451.1
MCU_VDD  (via drill 0.3)
  Top 0.152: U0101.32 72.66,14.97 72.39,15.56 v71.75,16.51 | U0101.19 66.16,15.67 v66.36,15.88 | U0101.64 65.16,23.11 v66.04,21.27 | L0411.1 58.74,15.24 v58.42,15.56
  Bottom 0.152: C0402.1 71.77,16.21 v71.75,16.51 71.75,18.73 71.44,19.05 SJ0401.2 | C0403.1 65.95,21.5 v66.04,21.27 66.04,20.95 66.67,20.32 68.99,20.32 69.42,19.89 | SJ0401.2 69.42,19.89 | 69.42,19.89 69.85,20.32 69.85,21.21 C0410.1 | SJ0401.2 69.42,17.99 67.31,15.88 v66.36,15.88 66.34,15.86 C0401.1 66.04,13.97 64.14,12.06 59.37,12.06 57.78,13.65 57.78,14.92 v58.42,15.56
MCU_VDDA  (via drill 0.3)
  Top 0.152: U0101.13 62.69,16.75 L0411.2 61.17,14.71 v61.28,14.61
  Bottom 0.152: C0413.1 60.82,14.14 v61.28,14.61 60.9,14.99 C0412.1
MCU_VREF_M
  Top 0.152: U0101.12 61.72,17.25 R0441.2
MP_CAT_CTS_R  (via drill 0.3)
  Top 0.152: U1101.10 36.2,13.02 36.83,13.65 46.35,13.65 47.62,14.92 47.62,25.4 47.94,25.72 v55.56,25.72
  Bottom 0.152: v55.56,25.72 R1103.2
MP_CAT_RTR_R
  Top 0.152: U1101.9 R1104.2
MP_CAT_RXD_R
  Top 0.152: U1101.11 37.47,12.7 37.78,13.02 44.45,13.02 45.09,12.38 58.74,12.38 59.05,12.06 59.05,10.79 R1101.2
MP_CAT_TXD_R
  Top 0.152: U1101.12 R1102.2
MP_RS_CTS_R  (via drill 0.3)
  Top 0.152: R1003.2 v82.55,14.92 | v82.87,40.96 83.19,41.27 U1001.10
  Bottom 0.152: v82.55,14.92 82.55,28.89 82.23,29.21 76.83,29.21 75.88,30.16 75.88,31.43 82.87,38.42 v82.87,40.96
MP_RS_RTR_R
  Top 0.152: U1001.9 86.68,40.01 87,39.69 R1004.2
MP_RS_RXD_R  (via drill 0.3)
  Top 0.152: U1001.11 83.82,42.55 83.19,43.18 v82.87,43.18 | v60.96,33.02 56.83,33.02 56.52,32.7 v56.52,22.23
  Bottom 0.152: v82.87,43.18 81.28,43.18 79.06,40.96 79.06,38.42 73.66,33.02 v60.96,33.02 | v56.52,22.23 59.05,19.68 R1001.2
MP_RS_TXD_R
  Top 0.152: U1001.12 86.68,43.81 87,43.5 R1002.2
N$12
  Top 0.152: U0601.22 33.38,58.48 R0611.2
N$13
  Top 0.152: U0701.22 49.88,58.48 R0711.2
N$15
  Top 0.152: U0801.22 66.39,58.48 R0811.2
PA0
  Top 0.152: U0101.14 64.22,16.19 62.87,16.19 62.23,15.56 62.23,14.61 62.87,13.97 62.87,13.34 62.55,13.02 61.28,13.02 60.96,12.7 60.96,11.11 60.64,10.79 R1101.1
PA1  (via drill 0.3)
  Top 0.152: U0101.15 63.38,15.75 v62.87,15.24 | R1102.1 v38.73,6.35 | v61.91,13.65 v47.62,13.65
  Bottom 0.152: v62.87,15.24 62.87,14.61 v61.91,13.65 | v47.62,13.65 46.04,13.65 v38.73,6.35
PA3
  Top 0.152: U0101.17 63.91,14.38 63.5,13.97 63.5,12.48 63.18,12.06 R0922.1
PA5
  Top 0.152: U0101.21 67.16,13.5 66.36,12.7 R0621.1
PA6  (via drill 0.3)
  Top 0.152: U0101.22 67.66,13.36 v67.46,13.02
  Bottom 0.152: R0622.1 v67.46,13.02
PA7
  Top 0.152: U0101.23 68.16,12.17 R0623.1
PA9  (via drill 0.3)
  Top 0.152: U0101.42 81.85,19.75 v85.09,16.51 | v88.27,18.73 88.39,19.05
  Top 0.305: X1401.VBUS 89.64,20.29 88.39,19.05 PF1411.1
  Bottom 0.152: v85.09,16.51 87.95,16.51 88.27,16.83 v88.27,18.73
PA10
  Top 0.152: X1401.ID 92.69,22.24 93.03,21.91 93.03,18.73 91.12,16.83 87.31,16.83 86.68,17.46 86.68,20 86.36,20.32 77.47,20.32 77.4,20.25 U0101.43
PA11
  Top 0.152: X1401.D- 76.5,20.94 76.31,20.75 U0101.44
PA12
  Top 0.152: X1401.D+ 76.2,21.59 75.86,21.25 U0101.45
PA13  (via drill 0.3)
  Top 0.152: U0101.46 74.77,21.75 v74.93,21.91
  Bottom 0.152: R0231.1 76.53,6.35 X0201.2 78.42,6.35 78.42,21.59 78.11,21.91 v74.93,21.91
PA14  (via drill 0.3)
  Top 0.152: U0101.49 72.84,23.62 73.34,24.13 v76.2,24.13
  Bottom 0.152: R0232.2 76.37,5.08 78.42,5.08 79.63,6.29 X0201.4 79.63,23.88 79.38,24.13 v76.2,24.13
PA15  (via drill 0.3)
  Top 0.152: U0101.50 72.07,23.71 v72.07,24.77
  Bottom 0.152: R1103.1 72.07,25.61 v72.07,24.77
PB0
  Top 0.152: U0101.26 69.66,13.46 69.53,12.7 R0624.1
PB1  (via drill 0.3)
  Top 0.152: U0101.27 70.16,13.16 70.17,13.02 v70.17,12.91
  Bottom 0.152: v70.17,12.91 R0724.1
PB2
  Top 0.152: U0101.28 70.66,13.48 71.12,12.38 R0824.1
PB6
  Top 0.152: X0601.1 76.83,27.3 72.72,27.3 R0512.1 72.71,27.62 72.39,27.94 69.22,27.94 68.9,27.62 68.9,25.08 68.16,24.34 U0101.58
PB7  (via drill 0.3)
  Top 0.152: U0101.59 67.63,23.65 67.63,24.45 67.94,24.77 v67.94,25.08 | v54.93,25.08 v48.58,25.08 | v46.67,25.08 42.23,25.08 v39.69,22.54 | R1104.1 v34.92,6.35
  Bottom 0.152: v67.94,25.08 v54.93,25.08 | v48.58,25.08 v46.67,25.08 | v34.92,6.35 34.92,17.78 v39.69,22.54
PB9  (via drill 0.3)
  Top 0.152: X0601.3 77.79,25.72 71.75,25.72 71.44,26.04 R0511.1 71.42,27.3 v69.85,27.3 | U0101.62 66.16,26.15 v66.36,26.35
  Bottom 0.152: v66.36,26.35 66.99,26.35 67.94,27.3 v69.85,27.3
PB10  (via drill 0.3)
  Top 0.152: U0101.29 71.16,13.62 72.71,12.06 v80.96,12.06 | v88.9,42.55 89.22,42.86 89.22,43.4 R1002.1
  Bottom 0.152: v80.96,12.06 80.96,24.45 80.64,24.77 76.83,24.77 74.61,26.99 74.61,32.7 80.33,38.42 80.33,40.96 81.6,42.23 88.58,42.23 v88.9,42.55
PB11
  Top 0.152: U0101.30 71.66,13.75 72.07,13.34 R0626.1
PB12
  Top 0.152: U0101.33 75.66,15.25 R1003.1
PB13  (via drill 0.3)
  Top 0.152: U0101.34 74.49,15.75 74.93,16.19 v81.6,16.19 | v88.9,40.64 89.22,40.32 89.22,39.79 R1004.1
  Bottom 0.152: v81.6,16.19 81.6,25.08 81.28,25.4 76.83,25.4 75.25,26.99 75.25,32.07 81.28,38.1 81.28,40.32 82.55,41.59 83.19,41.59 84.14,40.64 v88.9,40.64
PC0  (via drill 0.3)
  Top 0.152: U0101.8 63.62,19.25 62.87,20 v62.87,20.32 | v55.56,24.45 v49.21,24.45
  Bottom 0.152: v62.87,20.32 62.87,24.13 62.55,24.45 v55.56,24.45 | v49.21,24.45 46.04,24.45 45.4,25.08 36.83,25.08 30.8,31.11 18.1,31.11 17.14,30.16 17.14,28.26 15.56,26.67 15.56,25.4 15.89,25.07 R0952.2
PC1  (via drill 0.3)
  Top 0.152: U0101.9 64.26,18.73 63.5,18.73 v62.23,19.68
  Bottom 0.152: R1001.1 v62.23,19.68
PC2  (via drill 0.3)
  Top 0.152: D0961.A 15.04,26.22 R0961.2 v16.19,26.04 | U0101.10 63.35,18.25 62.87,18.41 61.91,19.05 61.59,19.37 61.59,20.32 v61.91,20.64 | v54.93,23.81 v48.58,23.81
  Bottom 0.152: v61.91,20.64 61.91,23.5 61.59,23.81 v54.93,23.81 | v48.58,23.81 43.81,23.81 43.18,24.45 36.2,24.45 30.16,30.48 18.41,30.48 18.1,30.16 18.1,27.94 v16.19,26.04
PC3
  Top 0.152: U0101.11 61.96,17.75 R0921.1
PC4  (via drill 0.3)
  Top 0.152: U0101.24 68.66,13.26 v68.9,13.02
  Bottom 0.152: R0625.1 v68.9,13.02
PC14_OSC32_IN
  Top 0.152: Q0321.2 58.12,23.97 | 58.12,23.97 C0331.- | 58.12,23.97 58.59,23.8 C0332.1 60.98,23.81 61.59,23.81 63.66,21.75 U0101.3
PC15_OSC32_OUT
  Top 0.152: U0101.4 63.5,21.25 61.59,21.57 60.96,21.57 Q0321.1 60.64,20 60.3,19.68 58.74,19.68 58.44,19.38 C0311.1
PH3_BOOT0
  Top 0.152: U0101.60 67.16,27.46 X0222.2
  Bottom 0.152: R0221.2 66.06,28.56 X0222.2
RELAY1
  Top 0.152: U0601.1 26.88,48.69 22.54,53.02 22.54,56.83 16.51,62.87 X1601.1
RELAY2
  Top 0.152: U0601.2 27.52,48.67 23.18,53.02 23.18,56.83 17.78,62.23 17.78,65.41 16.51,66.67 X1601.2
RELAY3
  Top 0.152: U0601.4 28.82,48.33 28.51,48.33 23.81,53.02 23.81,56.83 19.05,61.59 X1601.3
RELAY4
  Top 0.152: U0601.5 29.48,48.63 29.21,48.9 28.57,48.9 24.45,53.02 24.45,56.83 20.32,60.96 20.32,65.41 19.05,66.67 X1601.4
RELAY5  (via drill 0.3)
  Top 0.152: U0601.12 34.02,48.31 v35.88,50.16
  Bottom 0.152: X1601.5 21.59,64.14 35.24,50.48 v35.88,50.16
RELAY6  (via drill 0.3)
  Top 0.152: U0601.13 34.67,48.33 35.56,49.21 35.88,49.21 36.51,49.85 v36.51,50.8
  Bottom 0.152: X1601.6 22.86,66.04 22.86,64.14 36.2,50.8 v36.51,50.8
RELAY7  (via drill 0.3)
  Top 0.152: U0601.15 35.98,48.36 37.15,49.53 v37.15,50.16
  Bottom 0.152: X1601.7 24.13,63.82 37.15,51.12 v37.15,50.16
RELAY8  (via drill 0.3)
  Top 0.152: U0601.16 36.62,48.05 37.78,49.21 v37.78,50.8
  Bottom 0.152: X1601.8 25.4,66.04 25.4,63.82 37.78,51.44 v37.78,50.8
RELAY9  (via drill 0.3)
  Top 0.152: U0601.17 36.62,57.58 36.72,57.9 v36.83,57.78
  Bottom 0.152: X1601.9 26.67,63.5 33.02,57.15 36.2,57.15 v36.83,57.78
RELAY10  (via drill 0.3)
  Top 0.152: U0601.18 35.98,58.2 v36.2,58.42
  Bottom 0.152: X1601.10 27.94,66.04 27.94,62.87 33.34,57.47 35.24,57.47 v36.2,58.42
RELAY11  (via drill 0.3)
  Top 0.152: U0601.20 34.67,58.17 34.92,58.42 v35.24,58.42
  Bottom 0.152: X1601.11 29.21,62.23 33.34,58.1 34.92,58.1 v35.24,58.42
RELAY12  (via drill 0.3)
  Top 0.152: U0601.21 34.02,58.47 v34.61,59.05
  Bottom 0.152: X1601.12 30.48,66.04 30.48,61.59 32.7,59.37 34.29,59.37 v34.61,59.05
RELAY13
  Top 0.152: U0601.28 29.48,61.23 31.75,63.5 X1601.13
RELAY14
  Top 0.152: U0601.29 28.82,61.53 30.48,63.18 30.48,66.04 X1601.14
RELAY15
  Top 0.152: X1601.15 33.02,66.04 33.02,68.26 32.7,68.58 28.26,68.58 27.94,68.26 27.94,62.55 27.52,62.13 U0601.31
RELAY16
  Top 0.152: U0601.32 26.88,62.44 25.4,63.82 25.4,68.9 25.72,69.22 33.97,69.22 34.29,68.9 X1601.16
RELAY17
  Top 0.152: X1601.17 36.83,60.96 39.37,58.42 39.37,52.7 43.38,48.69 U0701.1
RELAY18
  Top 0.152: U0701.2 44.03,48.67 40.01,52.7 40.01,58.42 38.1,60.33 38.1,66.04 X1601.18
RELAY19
  Top 0.152: X1601.19 39.37,59.69 40.64,58.42 40.64,52.7 45.09,48.26 45.4,48.26 45.4,47.49 U0701.4
RELAY20
  Top 0.152: U0701.5 45.98,48.63 45.72,48.9 45.09,48.9 41.27,52.7 41.27,58.42 40.96,58.74 40.96,65.09 39.37,66.67 X1601.20
RELAY21
  Top 0.152: U0701.12 50.53,48.31 57.15,54.93 X1602.1
RELAY22
  Top 0.152: U0701.13 51.19,48.33 57.78,54.93 57.78,63.5 58.42,64.14 58.42,66.04 X1602.2
RELAY23
  Top 0.152: U0701.15 52.48,48.36 58.42,54.29 58.42,62.23 59.69,63.5 X1602.3
RELAY24
  Top 0.152: U0701.16 53.13,48.37 59.05,54.29 59.05,61.91 60.96,63.82 60.96,66.04 X1602.4
RELAY25  (via drill 0.3)
  Top 0.152: U0701.17 53.13,57.58 v53.34,57.78
  Bottom 0.152: X1602.5 60.96,66.04 60.96,68.26 60.64,68.58 53.66,68.58 53.34,68.26 v53.34,57.78
RELAY26  (via drill 0.3)
  Top 0.152: U0701.18 52.48,58.2 v52.7,58.42
  Bottom 0.152: X1602.6 62.23,68.9 61.91,69.22 53.02,69.22 52.7,68.9 v52.7,58.42
RELAY27  (via drill 0.3)
  Top 0.152: U0701.20 51.19,57.85 v51.75,58.42
  Bottom 0.152: X1602.7 63.5,66.04 63.5,69.53 63.18,69.85 52.07,69.85 51.75,69.53 v51.75,58.42
RELAY28  (via drill 0.3)
  Top 0.152: U0701.21 50.53,58.47 v51.12,59.05
  Bottom 0.152: X1602.8 64.77,70.17 64.45,70.48 51.44,70.48 51.12,70.17 v51.12,59.05
RELAY29
  Top 0.152: X1602.9 66.04,66.04 66.04,68.26 65.72,68.58 46.35,68.58 45.98,68.21 U0701.28
RELAY30
  Top 0.152: X1602.10 67.31,68.9 66.99,69.22 45.72,69.22 45.34,68.83 U0701.29
RELAY31
  Top 0.152: X1602.11 68.58,66.04 68.58,69.53 68.26,69.85 44.45,69.85 44.03,69.44 U0701.31
RELAY32
  Top 0.152: X1602.12 69.85,70.17 69.53,70.48 43.81,70.48 43.38,70.06 U0701.32
RELAY33  (via drill 0.3)
  Top 0.152: U0801.1 57.99,47.42 v57.78,47.62
  Bottom 0.152: v57.78,47.62 56.52,47.62 56.2,47.94 56.2,50.8 59.69,54.29 72.07,54.29 72.39,54.61 X1602.13
RELAY34  (via drill 0.3)
  Top 0.152: U0801.2 60.55,48.36 60.33,48.58 v58.42,48.58
  Bottom 0.152: v58.42,48.58 57.15,48.58 56.83,48.9 56.83,50.48 60.01,53.66 73.34,53.66 73.66,53.98 73.66,66.04 X1602.14
RELAY35  (via drill 0.3)
  Top 0.152: U0801.4 61.84,48.01 60.64,49.21 v57.78,49.21
  Bottom 0.152: v57.78,49.21 57.47,49.53 57.47,50.16 60.33,53.02 74.61,53.02 74.93,53.34 X1602.15
RELAY36  (via drill 0.3)
  Top 0.152: U0801.5 62.49,48.63 62.23,48.9 61.59,48.9 60.64,49.85 v58.42,49.85
  Bottom 0.152: v58.42,49.85 60.96,52.39 75.88,52.39 76.2,52.7 76.2,66.04 X1602.16
RM_FWD
  Bottom 0.305: X1501.1 L0901.2
RM_REV
  Bottom 0.152: L0911.2 X1511.1
RS_DTE_CTS
  Top 0.152: U1001.7 81.6,41.27 81.92,40.96 81.92,38.73 82.55,38.1 X1053.1
  Bottom 0.152: C1053.1 91.86,38.95 X1053.1
RS_DTE_RTR
  Top 0.152: U1001.8 80.01,39.95 80.01,38.1 85.09,33.02 X1053.2
  Bottom 0.152: C0054.1 91.86,33.87 X1053.2
RS_DTE_RXD  (via drill 0.3)
  Top 0.152: v88.27,46.35 U1001.14
  Bottom 0.152: v88.27,46.35 88.9,46.99 88.9,60.33 89.53,60.96 X1051.1 91.86,61.81 C1051.1
RS_DTE_TXD  (via drill 0.3)
  Top 0.152: v88.9,45.09 U1001.13
  Bottom 0.152: v88.9,45.09 90.17,46.35 90.17,55.24 90.81,55.88 X1051.2 91.86,56.73 C1052.1
RS_MX_C1N1
  Top 0.152: U1001.3 78.74,46.35 77.47,47.62 76.84,47.62 C1002.2
RS_MX_C1P
  Top 0.152: U1001.1 78.42,48.9 77.79,49.53 76.84,49.53 C1002.1
RS_MX_C2M1
  Top 0.152: U1001.5 78.11,43.81 77.79,43.5 76.84,43.5 C1003.2
RS_MX_C2P
  Top 0.152: U1001.4 78.11,45.09 77.79,45.4 76.84,45.4 C1003.1
RS_MX_VM
  Top 0.152: U1001.6 78.74,42.55 77.47,41.27 77.15,41.27 C1005.1
RS_MX_VP
  Top 0.152: U1001.2 81.28,47.62 81.6,47.94 81.6,49.53 81.28,49.85 80.01,49.85 79.69,50.16 79.69,51.12 C1004.1
SPI_DRV_!RST  (via drill 0.3)
  Top 0.152: U0701.27 46.63,61.88 v46.67,61.91 v54.61,61.91 | U0801.27 63.15,61.88 v63.18,61.91 72.71,61.91 73.03,61.59 v73.03,42.86 | U0601.27 30.12,59.65 v32.38,61.91 | v61.28,36.2 v51.75,36.2
  Bottom 0.152: v46.67,61.91 v32.38,61.91 | v54.61,61.91 v63.18,61.91 | v73.03,42.86 73.03,39.37 69.85,36.2 v61.28,36.2 | R0625.2 68.9,8.57 67.94,7.62 65.09,7.62 64.45,8.26 56.83,8.26 52.07,13.02 52.07,35.88 v51.75,36.2
SPI_DRV_C_!CS  (via drill 0.3)
  Top 0.152: v50.16,39.69 50.48,40.01 v62.23,40.01 | v60.33,41.59 53.98,41.59 51.84,43.73 U0701.14
  Bottom 0.152: R0724.2 70.48,7.62 69.22,6.35 64.45,6.35 63.82,6.99 56.2,6.99 50.8,12.38 50.8,35.24 50.16,35.88 v50.16,39.69 | v62.23,40.01 62.23,41.27 61.91,41.59 v60.33,41.59
SPI_DRV_EXT_!CS  (via drill 0.3)
  Top 0.152: R0824.2 v71.12,9.53 | U0801.14 68.34,45.95 70.17,44.13 v70.17,42.86 | v60.33,38.1 v49.21,38.1
  Bottom 0.152: v71.12,9.53 71.12,6.99 69.85,5.71 64.14,5.71 63.5,6.35 55.88,6.35 50.16,12.06 50.16,34.92 49.21,35.88 v49.21,38.1 | v70.17,42.86 70.17,39.37 68.9,38.1 v60.33,38.1
SPI_DRV_L_!CS  (via drill 0.3)
  Top 0.152: U0601.14 35.33,45.95 35.88,45.4 v35.88,43.81 | R0624.2 v69.53,9.53 | v61.28,38.73 v50.8,38.73
  Bottom 0.152: v35.88,43.81 44.13,43.81 45.09,44.77 51.44,44.77 52.39,43.81 60.64,43.81 61.59,44.77 66.67,44.77 69.53,42.23 69.53,39.69 68.58,38.73 v61.28,38.73 | v69.53,9.53 69.53,7.94 68.58,6.99 64.77,6.99 64.14,7.62 56.52,7.62 51.44,12.7 51.44,35.56 50.8,36.2 v50.8,38.73
SPI_DRV_PWM  (via drill 0.3)
  Top 0.152: v44.77,61.28 44.69,61.2 U0701.30 44.69,55.8 v42.86,53.98 | U0801.30 61.2,61.2 v61.28,61.28 | v47.94,61.28 v55.56,61.28 | U0601.30 28.18,55.33 v28.26,55.24 | v69.85,61.28 72.07,61.28 72.39,60.96 72.39,45.4 v72.07,45.09 | R0626.2 v83.5,13.34 | v77.47,38.1 v83.5,32.07 | v88.9,29.21 v83.5,23.81
  Bottom 0.152: v44.77,61.28 v47.94,61.28 | v55.56,61.28 v61.28,61.28 v69.85,61.28 | v42.86,53.98 38.1,49.21 35.56,49.21 29.53,55.24 v28.26,55.24 | v72.07,45.09 73.66,43.5 73.66,39.37 73.98,39.05 77.15,39.05 77.47,38.73 v77.47,38.1 | v83.5,13.34 v83.5,23.81 | v83.5,32.07 86.04,32.07 v88.9,29.21
SPI_DRV_SCLK  (via drill 0.3)
  Top 0.152: U0601.11 33.38,46.63 34.61,45.4 v34.61,43.18 | U0701.11 49.88,46.63 51.12,45.4 v51.12,43.18 | U0801.11 66.39,46.63 68.9,44.13 v68.9,41.91 | R0621.2 v66.36,9.53 | v54.61,39.37 v60.33,39.37
  Bottom 0.152: v34.61,43.18 44.45,43.18 45.4,44.13 50.16,44.13 v51.12,43.18 60.96,43.18 61.91,44.13 66.36,44.13 v68.9,41.91 68.9,40.01 68.26,39.37 v60.33,39.37 | v66.36,9.53 65.72,10.16 57.78,10.16 53.98,13.97 53.98,34.61 54.61,35.24 v54.61,39.37
SPI_DRV_SI  (via drill 0.3)
  Top 0.152: U0701.19 51.84,55.48 v52.39,54.93 | U0801.19 68.34,55.8 v68.9,55.24 70.8,53.34 v70.8,41.91 | U0601.19 35.33,55.48 v35.88,54.93 | R0623.2 v67.94,9.53 | v61.28,37.47 v52.7,37.47
  Bottom 0.152: v68.9,55.24 68.58,54.93 v52.39,54.93 v35.88,54.93 | v70.8,41.91 70.8,39.05 69.22,37.47 v61.28,37.47 | v67.94,9.53 67.94,8.89 67.31,8.26 65.41,8.26 64.77,8.89 57.15,8.89 52.7,13.34 v52.7,37.47
SPI_DRV_SO  (via drill 0.3)
  Top 0.152: v54.29,60.33 54.19,60.22 R0711.1 48.16,60.22 v47.94,60.33 | v65.09,60.33 65.94,59.91 R0811.1 71.22,60.02 71.44,59.69 v71.44,42.86 | R0611.1 35.46,60.22 v35.56,60.33 | v60.33,36.83 v53.66,36.83
  Bottom 0.152: v54.29,60.33 v65.09,60.33 | v35.56,60.33 v47.94,60.33 | v71.44,42.86 71.44,38.73 69.53,36.83 v60.33,36.83 | R0622.2 67.31,9.21 66.99,8.89 65.72,8.89 65.09,9.53 57.47,9.53 53.34,13.65 53.34,36.51 v53.66,36.83
SWR_IN_FWD  (via drill 0.3)
  Top 0.152: D0901.A 4.76,24.24 4.76,25.08 6.35,26.67 R0903.1 6.97,26.05 v7.3,25.72
  Bottom 0.152: R0902.2 7.62,25.4 v7.3,25.72 4.8,28.22 U0921.1
SWR_IN_FWD_HI
  Bottom 0.305: C0901.1 5.93,22.64 6.35,22.23 L0901.1 | C0901.1 R0901.2 | C0901.1 7.2,22.86 R0902.1
SWR_IN_REV  (via drill 0.3)
  Top 0.152: D0911.A 8.05,32.5 v7.3,31.75 8.24,30.81 R0913.1
  Bottom 0.152: R0912.2 7.62,32.07 v7.3,31.75 7.9,31.15 U0921.5
SWR_IN_REV_HI
  Bottom 0.152: C0911.1 5.73,34.62 6.35,35.24 L0911.1 | R0912.1 6.97,33.67 6.35,34.29 C0911.1 | R0911.2 C0911.1
SWR_OP_OUT  (via drill 0.3)
  Top 0.152: D0951.C 12.7,25.08 13.02,24.77 v14.61,24.77
  Bottom 0.152: R0952.1 14.07,23.18 13.97,23.18 13.64,23.51 U0951.1 14.58,24.74 v14.61,24.77
SWR_SEL_FWD  (via drill 0.3)
  Top 0.152: R0921.2 60.33,18.11 60.33,18.73 50.16,18.73 v48.58,20.32 | v9.21,28.57 12.06,28.57 12.38,28.89 18.73,28.89 v19.05,28.57
  Bottom 0.152: v48.58,20.32 47.62,21.27 43.18,21.27 41.27,23.18 34.92,23.18 29.53,28.57 v19.05,28.57 | U0921.7 8.82,28.96 v9.21,28.57
SWR_SEL_PWR  (via drill 0.3)
  Top 0.152: D0951.A v12.7,27.94
  Bottom 0.152: v12.7,27.94 12.09,27.33 U0951.4 11.76,28.25 11.43,28.57 11.43,29.2 R0951.2 11.16,29.46 U0921.6 6.6,29.46 6.1,28.96 U0921.2
SWR_SEL_REV  (via drill 0.3)
  Top 0.152: R0922.2 60.31,12.08 59.37,13.02 v49.45,13.02 | v6.03,30.16 6.67,29.53 v20,29.53
  Bottom 0.152: v49.45,13.02 49.45,20.4 47.62,22.23 43.81,22.23 42.23,23.81 35.56,23.81 29.84,29.53 v20,29.53 | U0921.3 5.08,29.53 5.4,29.53 v6.03,30.16
TPS_LBI  (via drill 0.3)
  Top 0.152: U1301.6 14.24,36.47 13.97,36.2 v13.32,36.2
  Bottom 0.152: R1302.1 v13.32,36.2 | 13.12,36.62 13.12,36.41
  Bottom 0.305: 13.12,36.62 R1301.2 | 13.12,36.41 v13.32,36.2
TPS_LBO  (via drill 0.3)
  Top 0.152: 15.74,42.41 17.14,43.81 23.5,43.81 24.77,42.55 v24.77,41.27
  Top 0.305: U1301.2 15.74,42.41
  Bottom 0.305: R1322.1 24.55,41.06 v24.77,41.27
TPS_PG  (via drill 0.3)
  Top 0.152: U1301.4 14.74,40.77 v13.65,39.69
  Bottom 0.152: R1321.1 24.55,39.27 v24.13,39.37 18.73,39.37 17.78,40.64 14.61,40.64 v13.65,39.69
TPS_SW
  Top 0.254: U1301.9 15.74,38.6 15.88,38.73
  Top 0.305: 15.88,38.73 17.24,38.73 18.73,36.83 L1311.4 L1311.2
USB_SHIELD
  Bottom 0.305: X1401.JSHIELD 93.36,19.09 X1401.JSHIELD@3 X1401.JSHIELD@4 X1401.JSHIELD@5 X1401.JSHIELD@6 93.36,24.11 X1401.JSHIELD@2 91.63,24.11 C1403.2 R1402.2
VDDUSB  (via drill 0.3)
  Top 0.152: U0101.48 84.88,22.75 v85.09,22.54 | v85.09,18.73 85.09,18.92 PF1411.2
  Bottom 0.152: v85.09,22.54 v85.09,18.73

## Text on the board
tPlace: 2 | 22 | 36 | 12V | 12V | DL0WH BiTuner Ctrl V1.0 / (C) 2019 | 23 | - | 1 | 21 | 22 | 35 | 12V | 12V | BAT | RELAY A | RELAY B | RXD | RS232 | TXD | 12V | + | GND | FWD | GND | CTS | BOOT0 | I2C | RTR | SCL | SDA | USB | REV | CAT Ifc. | SWD | RTR | CTS | GND | GND | TXD | RXD | RESET
Measures: 4x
